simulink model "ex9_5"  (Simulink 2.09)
settings: Solver=ode45  StartTime=0.0  StopTime=100.0  RelTol=1e-3  AbsTol=1e-6
undefined symbols (not defined in the file or in its folder): prog_bar

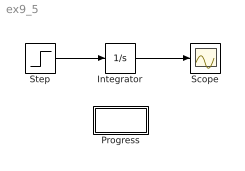
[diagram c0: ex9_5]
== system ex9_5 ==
  Integrator : Integrator  ExternalReset=none  InitialConditionSource=internal  InitialCondition=0  LimitOutput=off  UpperSaturationLimit=inf  LowerSaturationLimit=-inf  ShowSaturationPort=off  ShowStatePort=off  AbsoluteTolerance=auto
  Progress : Subsystem  Tag=prog_bar  mask{h_slider=292.000732421875}
      mask prompts: h_slider "Bar Handle"
  Scope : Scope
  Step : Step  Tag=prog_bar  Time=1  Before=0  After=1
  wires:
  Step/1 -> Integrator/1
  Integrator/1 -> Scope/1

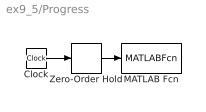
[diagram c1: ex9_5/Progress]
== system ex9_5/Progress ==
  Clock : Clock
  MATLAB Fcn : MATLABFcn  MATLABFcn=prog_bar('UpdateTime',h_slider,u(1))  OutputWidth=0
  Zero-Order Hold : ZeroOrderHold  SampleTime=.5
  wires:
  Clock/1 -> Zero-Order Hold/1
  Zero-Order Hold/1 -> MATLAB Fcn/1
